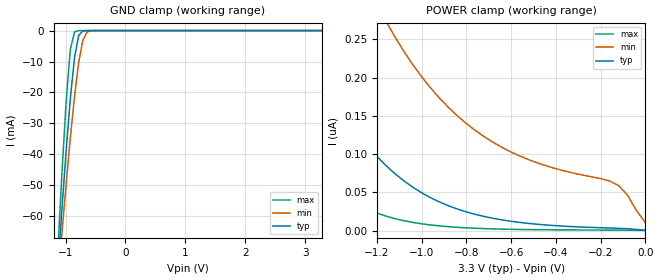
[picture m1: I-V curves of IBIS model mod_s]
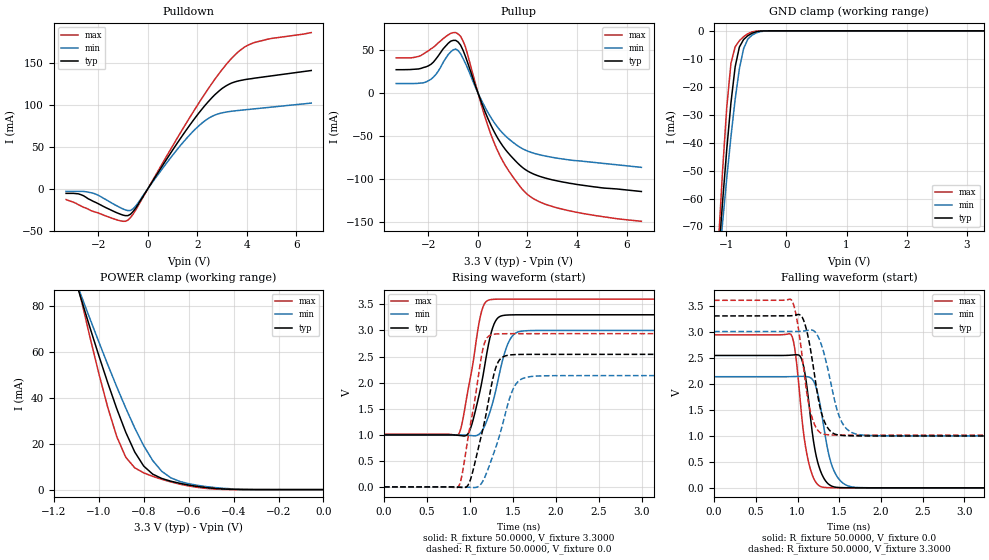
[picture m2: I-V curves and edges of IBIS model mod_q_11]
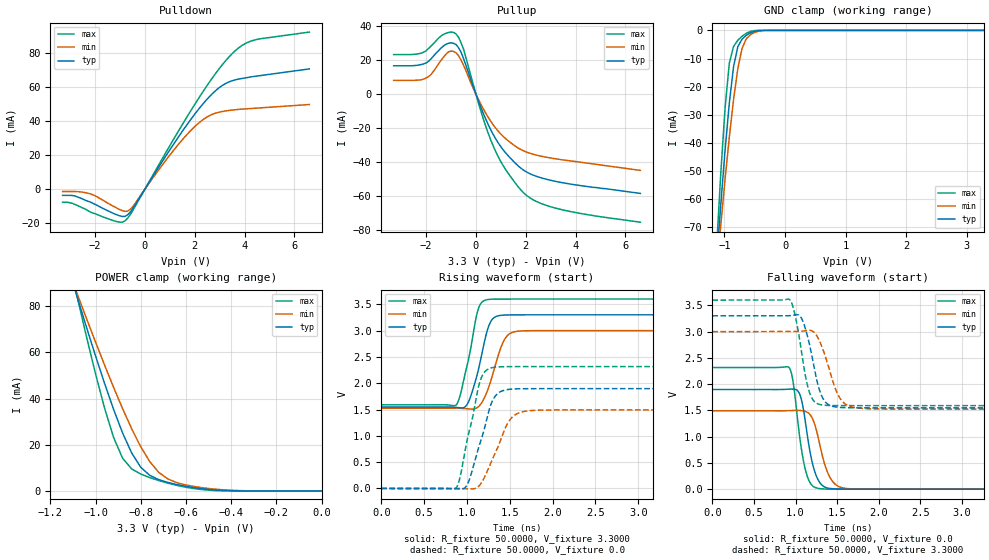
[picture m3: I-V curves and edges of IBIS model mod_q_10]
| IBIS (I/O, Buffer, Information, Specification) Model, officially
| electronic behavioral standard for Buffer structures of digital pins.
[IBIS ver]  4.0
[File name] pe_33_m95p32_3d3.ibs
[File Rev]  1.0
[Date]   13 December 2024
[Source]   CAD & Design Services (Catania) - STMicroelectronics
[Notes]
   (Note1)  This IBIS model includes the SO8N package parasitic data
   (Note2)  Pin 2 (S) and Pin 3,5,7 (WO2,DO0,HO3) have four driver
   stength cases: High, Medium, Qlow, Low;
   (Note3)  This IBIS model has some Notes about the non-monotonicity
   of the I-V curves, but they are not indicative of problems
   inside the model;
[Disclaimer]
   Customers are solely responsible for all aspects of their
   own product designs or applications using this IBIS Model.
   STMicroelectronics assumes no liability for Custmer Designs
   and applications associated to this IBIS Model.
   In the use of this IBIS Model Customer shall not modify,
   disassemble, alter this Model in whole or in part.
   If Customers do not accept these terms, the IBIS Model
   may not be used. For any problems or modifications please
   contact STMicroelectronics (www.st.com).
[Copyright] (c) 2024 STMicroelectronics
|   Component M95P32
[Component] M95P32
[Manufacturer] STMicroelectronics
[Package]
| variable   typ   min   max
R_pkg   0.0   0.0   0.0
L_pkg   0.0H   0.0H   0.0H
C_pkg   0.0F   0.0F   0.0F
[Pin]  signal_name   model_name   R_pin   L_pin   C_pin
1   S   mod_s   129.1m   2.1741nH   1.0266pF
2   QO1   mod_q   89.7m   1.6160nH   0.3359pF
3   WO2   mod_dwh   91.2m   1.6289nH   0.3576pF
4   VSS   GND   130.9m   2.1824nH   0.2874pF
5   DO0   mod_dwh   130.7m   2.1818nH   0.2862pF
6   C   mod_c   85.3m   1.5892nH   0.3544pF
7   HO3   mod_dwh   84.5m   1.5827nH   0.3547pF
8   VDD   POWER   124.1m   2.1422nH   0.2841pF
[Model Selector]   mod_q
mod_q_11   High drive: bit0='1', bit1='1'
mod_q_10   Med drive:  bit0='1', bit1='0'
mod_q_01   Qlow drive: bit0='0', bit1='1'
mod_q_00   Low drive:  bit0='0', bit1='0'
[Model Selector]   mod_dwh
mod_dwh_11   High drive: bit0='1', bit1='1'
mod_dwh_10   Med drive:  bit0='1', bit1='0'
mod_dwh_01   Qlow drive: bit0='0', bit1='1'
mod_dwh_00   Low drive:  bit0='0', bit1='0'
| Models and submodels in the file (10): mod_s (Input), mod_q_11 (Output), mod_q_10 (Output), mod_q_01 (Output), mod_q_00 (Output), mod_c (Input), mod_dwh_11 (I/O), mod_dwh_10 (I/O), mod_dwh_01 (I/O), mod_dwh_00 (I/O)
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|   Model mod_s
[Model]   mod_s
Model_type Input
Vinl   =  1.000V
Vinh   =  2.300V
C_comp   1.030pF   0.988pF   1.160pF
[Model Spec]
Vinl   1.000V  0.900V  1.080V  | <- for Vcc = 3.3V, 3.0V, 3.6V
Vinh   2.300V  2.100V  2.520V  | <- for Vcc = 3.3V, 3.0V, 3.6V
[Temperature Range]  25.0000   85.0000   -40.0000
[Voltage Range]   3.3000V   3.0000V   3.6000V
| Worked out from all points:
|   GND clamp passes 1 mA (typ) near -0.75 V on its own axis
[GND_clamp]
|Voltage   I(typ)   I(min)   I(max)
-3.3V     -780mA     -653.1mA   -1.006A
-1.13V    -77.77mA   -82.09mA   -71.95mA
-1.06V    -57.77mA   -65.56mA   -46.11mA
-990mV    -38.95mA   -49.68mA   -23.07mA
-920mV    -22.07mA   -34.75mA   -6.129mA
-850mV    -8.689mA   -21.3mA    -404.3uA
-780mV    -1.564mA   -10.23mA   -13.12uA
-710mV    -126.9uA   -3.043mA   -406.3nA
-640mV    -8.484uA   -469.3uA   -12.92nA
-570mV    -558.2nA   -52uA      -501pA
3.28V     283.4pA    72.53nA    27.68pA
[POWER_clamp]
|Voltage   I(typ)   I(min)   I(max)
-3.28V    4.906uA    5.748uA    3.96uA
-1.84V    554.1nA    960nA      271.9nA
-1.68V    381.2nA    730.9nA    162.8nA
-1.52V    252.1nA    547.5nA    90.84nA
-1.36V    159.8nA    404.6nA    47.05nA
-1.16V    85.18nA    274nA      18.97nA
-1.12V    74.57nA    253.4nA    15.71nA
-960mV    43.02nA    186.4nA    7.38nA
-760mV    21.2nA     130.8nA    3.054nA
-520mV    9.337nA    92.45nA    1.338nA
-120mV    3.038nA    58.93nA    663.6pA
0V        526.8pA    10.26nA    181.6pA
|   Model mod_q_11
[Model]   mod_q_11
Model_type Output
Polarity   Non-Inverting
Enable   Active-High
Vmeas   =  1.650V
Cref   =  30pF
C_comp   1.400pF   1.337pF   1.466pF
[Model Spec]
Vmeas  1.650V  1.500V  1.800V  | <- for Vcc = 3.3V, 3.0V, 3.6V
[Temperature Range]   25.0000   0.1050k   -40.0000
[Voltage Range]   3.3000V   3.0000V   3.6000V
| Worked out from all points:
|   slope of the pulldown table from 0 to 0.495 V, typ, clamps not added: 21.3 ohm
|   slope of the pullup table from 0 to 0.495 V, typ, clamps not added: 13.8 ohm
|   GND clamp passes 1 mA (typ) near -0.58 V on its own axis
|   POWER clamp passes 1 mA (typ) near -0.53 V on its own axis
|   rising waveform, R_fixture 50.0000, V_fixture 3.3000: 20-80 % time 167ps typ, 185ps min, 156ps max; typ from 0.995 V to 3.3 V
|   rising waveform, R_fixture 50.0000, V_fixture 0.0: 20-80 % time 197ps typ, 233ps min, 174ps max; typ from 0 V to 2.54 V
|   falling waveform, R_fixture 50.0000, V_fixture 0.0: 20-80 % time 135ps typ, 155ps min, 128ps max; typ from 2.54 V to 0 V
|   falling waveform, R_fixture 50.0000, V_fixture 3.3000: 20-80 % time 149ps typ, 180ps min, 137ps max; typ from 3.3 V to 0.995 V
[Pulldown]
|Voltage   I(typ)   I(min)   I(max)
-3.3V     -5.4mA     -3mA       -12.82mA
-2.8V     -6mA       -3mA       -19mA
-2.2V     -15mA      -5.3mA     -27mA
-1.2V     -29.2mA    -21.1mA    -37.6mA
-800mV    -32.02mA   -26.05mA   -37.38mA
-500mV    -23.51mA   -20.95mA   -25.93mA
1V        46.29mA    40.16mA    51.22mA
2V        88.39mA    73.76mA    99.86mA
2.6V      109.4mA    86.84mA    126.6mA
3.4V      126.8mA    92.92mA    156.7mA
4.3V      132.4mA    95.71mA    175mA
6.6V      141.6mA    102.6mA    187mA
[Pullup]
|Voltage   I(typ)   I(min)   I(max)
-3.3V     26.92mA    10.78mA    40.59mA
-2.5V     27.54mA    10.88mA    41.66mA
-2V       31.42mA    14.02mA    48.88mA
-1.1V     60.1mA     47.6mA     69.21mA
-800mV    59.17mA    49.22mA    68.51mA
-500mV    42.04mA    34.06mA    53.16mA
200mV     -15.63mA   -11.97mA   -20.15mA
700mV     -47.77mA   -36.41mA   -61.37mA
1.2V      -69.34mA   -52.57mA   -89.03mA
1.9V      -89.18mA   -66.58mA   -115.7mA
3.2V      -102.6mA   -76.15mA   -134.1mA
6.6V      -115mA     -86.85mA   -149.7mA
[GND_clamp]
|Voltage   I(typ)   I(min)   I(max)
-3.3V     -807.6mA   -672mA     -1.053A
-1.13V    -81.94mA   -85.75mA   -76.94mA
-1.06V    -61.58mA   -68.96mA   -50.51mA
-990mV    -42.58mA   -52.9mA    -27.53mA
-920mV    -25.81mA   -37.91mA   -11.64mA
-850mV    -12.88mA   -24.52mA   -5.709mA
-780mV    -5.82mA    -13.61mA   -3.523mA
-710mV    -3.106mA   -6.377mA   -2.091mA
-640mV    -1.742mA   -2.986mA   -1.046mA
-500mV    -309.6uA   -721.8uA   -69.16uA
-290mV    -791nA     -10.61uA   -17.06nA
3.28V     561.4pA    18.21uA    173.1pA
[POWER_clamp]
|Voltage   I(typ)   I(min)   I(max)
-3.28V    853.2mA    705.5mA    1.123A
-1.08V    83.64mA    85.1mA     83.66mA
-1V       58.53mA    64.51mA    50.75mA
-960mV    46.59mA    54.53mA    35.87mA
-920mV    35.3mA     44.85mA    23.13mA
-880mV    25.04mA    35.59mA    14.12mA
-840mV    16.42mA    26.93mA    9.512mA
-800mV    10.26mA    19.14mA    7.302mA
-720mV    4.876mA    8.001mA    4.493mA
-640mV    2.758mA    3.578mA    2.397mA
-400mV    94.29uA    284.7uA    12.64uA
0V        840.7pA    17.31nA    345.8pA
[Ramp]
| variable   typ   min   max
dV/dt_r   1.5248/0.2164n   1.2991/0.2403n   1.7626/0.1812n
dV/dt_f   1.3827/0.1694n   1.2128/0.2091n   1.5533/0.1622n
R_load = 50.0000
[Rising Waveform]
R_fixture= 50.0000
V_fixture= 3.3000
V_fixture_min= 3.0000
V_fixture_max= 3.6000
|time   V(typ)   V(min)   V(max)
0s        995.5mV    997.2mV    1.011V
864ps     988.9mV    997.8mV    1.002V
912ps     979.5mV    995.5mV    1.245V
1.008ns   1.127V     985mV      2.12V
1.136ns   1.991V     1.063V     3.371V
1.232ns   2.858V     1.436V     3.588V
1.312ns   3.217V     1.934V     3.599V
1.424ns   3.294V     2.672V     3.6V
1.584ns   3.3V       2.981V     3.6V
6ns       3.3V       3V         3.6V
[Rising Waveform]
R_fixture= 50.0000
V_fixture= 0.0
V_fixture_min= 0.0
V_fixture_max= 0.0
|time   V(typ)   V(min)   V(max)
0s        4.444nV    483.6nV    774.5pV
864ps     -5.061mV   869.7uV    -1.841mV
912ps     -12.78mV   -492.7uV   264mV
1.008ns   149.2mV    -8.221mV   1.222V
1.152ns   1.117V     115.5mV    2.655V
1.248ns   1.93V      511.3mV    2.916V
1.344ns   2.436V     985mV      2.936V
1.488ns   2.534V     1.823V     2.938V
1.664ns   2.541V     2.104V     2.938V
6ns       2.541V     2.133V     2.938V
[Falling Waveform]
R_fixture= 50.0000
V_fixture= 0.0
V_fixture_min= 0.0
V_fixture_max= 0.0
|time   V(typ)   V(min)   V(max)
0s        2.541V     2.133V     2.938V
920ps     2.548V     2.135V     2.949V
968ps     2.553V     2.137V     2.663V
1.048ns   2.478V     2.141V     1.408V
1.112ns   1.95V      2.135V     649.3mV
1.208ns   737.4mV    1.996V     137.7mV
1.288ns   274mV      1.44V      18.64mV
1.432ns   21.11mV    346.3mV    1.627mV
1.656ns   1.059mV    17.74mV    69.28uV
6ns       1.679uV    2.784uV    1.697uV
[Falling Waveform]
R_fixture= 50.0000
V_fixture= 3.3000
V_fixture_min= 3.0000
V_fixture_max= 3.6000
|time   V(typ)   V(min)   V(max)
0s        3.3V       3V         3.6V
928ps     3.304V     2.999V     3.607V
1.008ns   3.328V     3.002V     3.09V
1.088ns   3.148V     3.013V     2.089V
1.184ns   2.38V      3.024V     1.299V
1.248ns   1.72V      2.901V     1.095V
1.312ns   1.314V     2.615V     1.03V
1.504ns   1.011V     1.355V     1.012V
1.712ns   997.1mV    1.029V     1.011V
6ns       995.5mV    997.2mV    1.011V
|   Model mod_q_10
[Model]   mod_q_10
Model_type Output
Polarity   Non-Inverting
Enable   Active-High
Vmeas   =  1.650V
Cref   =  30pF
C_comp   1.400pF   1.337pF   1.466pF
[Model Spec]
Vmeas  1.650V  1.500V  1.800V  | <- for Vcc = 3.3V, 3.0V, 3.6V
[Temperature Range]   25.0000   0.1050k   -40.0000
[Voltage Range]   3.3000V   3.0000V   3.6000V
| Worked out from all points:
|   slope of the pulldown table from 0 to 0.495 V, typ, clamps not added: 42.6 ohm
|   slope of the pullup table from 0 to 0.495 V, typ, clamps not added: 27.6 ohm
|   GND clamp passes 1 mA (typ) near -0.58 V on its own axis
|   POWER clamp passes 1 mA (typ) near -0.53 V on its own axis
|   rising waveform, R_fixture 50.0000, V_fixture 3.3000: 20-80 % time 156ps typ, 173ps min, 148ps max; typ from 1.55 V to 3.3 V
|   rising waveform, R_fixture 50.0000, V_fixture 0.0: 20-80 % time 196ps typ, 232ps min, 174ps max; typ from 0 V to 1.9 V
|   falling waveform, R_fixture 50.0000, V_fixture 0.0: 20-80 % time 127ps typ, 153ps min, 118ps max; typ from 1.9 V to 0 V
|   falling waveform, R_fixture 50.0000, V_fixture 3.3000: 20-80 % time 148ps typ, 185ps min, 131ps max; typ from 3.3 V to 1.55 V
[Pulldown]
|Voltage   I(typ)   I(min)   I(max)
-3.3V     -3.6mA     -1.32mA    -7.7mA
-2.9V     -3.7mA     -1.32mA    -8.34mA
-2.2V     -7.5mA     -2.7mA     -13.3mA
-1.2V     -14.6mA    -10.5mA    -18.8mA
-800mV    -16.01mA   -13.02mA   -18.69mA
-500mV    -11.75mA   -10.47mA   -12.96mA
1V        23.15mA    20.08mA    25.61mA
2V        44.19mA    36.88mA    49.93mA
2.8V      57.58mA    44.65mA    67.43mA
3.5V      63.91mA    46.64mA    79.85mA
4.4V      66.5mA     47.7mA     87.91mA
6.6V      70.9mA     49.94mA    92.6mA
[Pullup]
|Voltage   I(typ)   I(min)   I(max)
-3.3V     16.6mA     8.02mA     23.18mA
-2.1V     17.69mA    8.788mA    24.57mA
-1.8V     20.64mA    11.45mA    28.17mA
-1.1V     29.8mA     24.81mA    36.14mA
-800mV    29.14mA    24.26mA    35.36mA
-500mV    21.02mA    17.03mA    26.58mA
200mV     -7.817mA   -5.983mA   -10.07mA
700mV     -23.89mA   -18.2mA    -30.68mA
1.2V      -34.67mA   -26.28mA   -44.52mA
1.9V      -44.59mA   -33.29mA   -57.84mA
3.3V      -51.61mA   -38.3mA    -67.42mA
6.6V      -58.4mA    -44.87mA   -75.3mA
[GND_clamp]
|Voltage   I(typ)   I(min)   I(max)
-3.3V     -807.6mA   -672mA     -1.053A
-1.13V    -81.94mA   -85.75mA   -76.94mA
-1.06V    -61.58mA   -68.96mA   -50.51mA
-990mV    -42.58mA   -52.9mA    -27.53mA
-920mV    -25.81mA   -37.91mA   -11.64mA
-850mV    -12.88mA   -24.52mA   -5.709mA
-780mV    -5.82mA    -13.61mA   -3.523mA
-710mV    -3.106mA   -6.377mA   -2.091mA
-640mV    -1.742mA   -2.986mA   -1.046mA
-500mV    -309.6uA   -721.8uA   -69.16uA
-290mV    -791nA     -10.61uA   -17.06nA
3.28V     561.4pA    18.21uA    173.1pA
[POWER_clamp]
|Voltage   I(typ)   I(min)   I(max)
-3.28V    853.2mA    705.5mA    1.123A
-1.08V    83.64mA    85.1mA     83.66mA
-1V       58.53mA    64.51mA    50.75mA
-960mV    46.59mA    54.53mA    35.87mA
-920mV    35.3mA     44.85mA    23.13mA
-880mV    25.04mA    35.59mA    14.12mA
-840mV    16.42mA    26.93mA    9.512mA
-800mV    10.26mA    19.14mA    7.302mA
-720mV    4.876mA    8.001mA    4.493mA
-640mV    2.758mA    3.578mA    2.397mA
-400mV    94.29uA    284.7uA    12.64uA
0V        840.7pA    17.31nA    345.8pA
[Ramp]
| variable   typ   min   max
dV/dt_r   1.1383/0.2199n   0.9181/0.2519n   1.3897/0.1890n
dV/dt_f   1.0516/0.1761n   0.8992/0.2300n   1.2059/0.1614n
R_load = 50.0000
[Rising Waveform]
R_fixture= 50.0000
V_fixture= 3.3000
V_fixture_min= 3.0000
V_fixture_max= 3.6000
|time   V(typ)   V(min)   V(max)
0s        1.547V     1.524V     1.59V
872ps     1.541V     1.525V     1.584V
920ps     1.533V     1.522V     1.766V
1.032ns   1.702V     1.511V     2.561V
1.128ns   2.222V     1.546V     3.392V
1.224ns   2.927V     1.799V     3.585V
1.288ns   3.2V       2.098V     3.597V
1.416ns   3.294V     2.759V     3.6V
1.576ns   3.3V       2.985V     3.6V
6ns       3.3V       3V         3.6V
[Rising Waveform]
R_fixture= 50.0000
V_fixture= 0.0
V_fixture_min= 0.0
V_fixture_max= 0.0
|time   V(typ)   V(min)   V(max)
0s        6.853nV    730.9nV    1.212nV
880ps     -4.601mV   520uV      22.21mV
928ps     -10.8mV    -684.4uV   276.5mV
1.008ns   88.88mV    -5.374mV   964.7mV
1.152ns   859.3mV    68.71mV    2.038V
1.216ns   1.219V     252mV      2.231V
1.296ns   1.661V     553.2mV    2.297V
1.504ns   1.886V     1.311V     2.316V
1.712ns   1.896V     1.475V     2.316V
6ns       1.897V     1.493V     2.316V
[Falling Waveform]
R_fixture= 50.0000
V_fixture= 0.0
V_fixture_min= 0.0
V_fixture_max= 0.0
|time   V(typ)   V(min)   V(max)
0s        1.897V     1.493V     2.316V
920ps     1.904V     1.495V     2.321V
968ps     1.905V     1.497V     2.075V
1.048ns   1.82V      1.499V     1.02V
1.112ns   1.356V     1.483V     414mV
1.192ns   573.2mV    1.381V     84.33mV
1.256ns   229.4mV    1.093V     21.45mV
1.4ns     17.32mV    267.8mV    1.5mV
1.592ns   1.056mV    17.33mV    67.99uV
6ns       1.915uV    2.763uV    2.005uV
[Falling Waveform]
R_fixture= 50.0000
V_fixture= 3.3000
V_fixture_min= 3.0000
V_fixture_max= 3.6000
|time   V(typ)   V(min)   V(max)
0s        3.3V       3V         3.6V
928ps     3.303V     2.999V     3.611V
992ps     3.316V     3V         3.331V
1.088ns   3.199V     3.009V     2.451V
1.184ns   2.641V     3.021V     1.777V
1.296ns   1.851V     2.796V     1.61V
1.376ns   1.632V     2.443V     1.595V
1.52ns    1.558V     1.77V      1.591V
1.712ns   1.548V     1.553V     1.59V
6ns       1.547V     1.524V     1.59V
